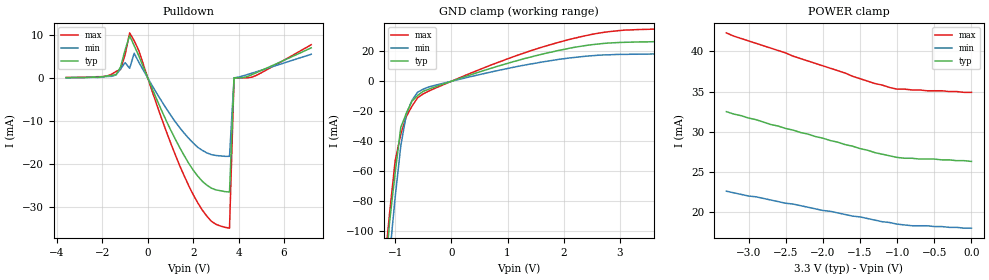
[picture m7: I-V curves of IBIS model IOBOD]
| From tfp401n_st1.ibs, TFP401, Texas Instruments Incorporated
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|   OPEN DRAIN INPUT / OUTPUT  MODEL
[Model]   IOBOD
Model_type   I/O_open_sink
| Signals   DFO
Vinl = 1.08
Vinh = 2.10
| variable   typ   min   max
C_comp   2pF   NA   NA
|   typ   min   max
[Temperature Range] 25.0   70.0   0.0
[Voltage range]   3.3V   3.0V   3.6V
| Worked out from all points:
|   GND clamp passes 1 mA (typ) near -0.08 V on its own axis
[GND_clamp]
|Voltage   I(typ)   I(min)   I(max)
-3.6V     -1.31A     -1.33A     -1.29A
-1.2V     -139mA     -162mA     -127mA
-1.1V     -94.5mA    -117mA     -88.5mA
-1V       -61.2mA    -77.6mA    -53.1mA
-900mV    -30.8mA    -43.2mA    -35.4mA
-800mV    -21.3mA    -21.8mA    -23.5mA
-700mV    -13.2mA    -12.7mA    -16.6mA
-600mV    -9.49mA    -7.29mA    -11mA
700mV     8.61mA     6.15mA     10.8mA
1.9V      20.6mA     14.6mA     26mA
2.7V      25.3mA     17.6mA     32.7mA
3.6V      26.5mA     18.3mA     34.9mA
[Power_clamp]
|Note that the [Power_clamp] voltage table is referenced to Vcc
|and is calculated using Vtable=Vcc-Vmeasured.
|Voltage   I(typ)   I(min)   I(max)
-3.3V     32.5mA     22.6mA     42.3mA
-3.2V     32.2mA     22.4mA     41.9mA
-2.5V     30.4mA     21.1mA     39.8mA
-2.4V     30.2mA     21mA       39.4mA
-1.7V     28.4mA     19.7mA     37.3mA
-1.6V     28.2mA     19.5mA     36.9mA
-1.3V     27.4mA     19mA       36mA
-1.1V     27mA       18.7mA     35.5mA
-1V       26.8mA     18.5mA     35.3mA
-800mV    26.7mA     18.3mA     35.2mA
-600mV    26.6mA     18.3mA     35.1mA
0V        26.3mA     18mA       34.9mA
[Pulldown]
|Voltage   I(typ)   I(min)   I(max)
-3.6V     102uA      74.8uA     124uA
-1.4V     804uA      728uA      1.54mA
-1.2V     2.59mA     2.11mA     1.99mA
-800mV    9.87mA     2.26mA     10.5mA
-600mV    7.53mA     5.77mA     8.67mA
1V        -12mA      -8.56mA    -15mA
2V        -21.4mA    -15.1mA    -27.1mA
2.8V      -25.6mA    -17.8mA    -33.3mA
3.6V      -26.5mA    -18.2mA    -34.9mA
3.8V      25.7uA     53.2uA     12.2uA
4.8V      1.29mA     1.49mA     667uA
7.2V      7.02mA     5.53mA     7.75mA
[Ramp]
|   typ   min   max
dV/dt_f   1.97v/0.51ns   1.78v/0.78ns   2.16v/0.36ns
dV/dt_r   1mv/1us   1mv/1us   1mv/1us
R_load = 5K
